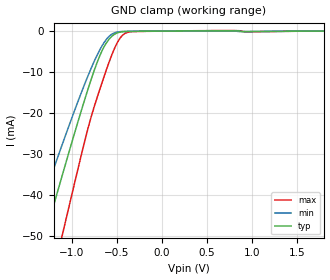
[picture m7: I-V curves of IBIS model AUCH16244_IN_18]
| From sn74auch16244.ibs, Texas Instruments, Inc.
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[Model]   AUCH16244_IN_18
Model_type  Input
Vinl=0.5775
Vinh=1.2675
| variable   typ   min   max
C_comp   3.43pF   2.61pF   4.05pF
[Temperature Range]   40   100   -40
| Ambient temperature   25   85   -40
[Voltage range]   1.8   1.65   1.95
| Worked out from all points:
|   GND clamp passes 1 mA (typ) near -0.54 V on its own axis
[GND Clamp]
| AUCH16244_IN_18
|   Voltage   I(typ)   I(min)   I(max)
-3.6V     -232.7mA   -194.4mA   -280.6mA
-1.44V    -61.25mA   -48.9mA    -81.22mA
-1.305V   -50.69mA   -40.25mA   -68.6mA
-1.265V   -47.59mA   -37.71mA   -64.86mA
-1.11V    -35.66mA   -28.03mA   -50.38mA
-1.06V    -31.86mA   -24.96mA   -45.71mA
-820mV    -14.33mA   -11.04mA   -23.92mA
-685mV    -5.94mA    -4.522mA   -14.1mA
-565mV    -1.53mA    -940.8uA   -6.488mA
-485mV    -387.3uA   -202.2uA   -2.536mA
-420mV    -131uA     -74.24uA   -760.5uA
1.8V      232pA      557.9nA    -933.9pA
